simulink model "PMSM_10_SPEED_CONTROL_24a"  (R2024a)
settings: Solver=ode45  StartTime=0.0  StopTime=0.2  MaxStep=1e-6  RelTol=1e-6  AbsTol=1e-6  EnableMultiTasking=on
undefined symbols (not defined in the file): by, established, Flux, linkage, magnets, V
libraries: spsIGBTDiodeLib x6, spsCurrentMeasurementLib x3, slpidlib x2, simulink x2, spsDCVoltageSourceLib x1, spsPermanentMagnetSynchronousMachineLib x1, spspowerguiLib x1

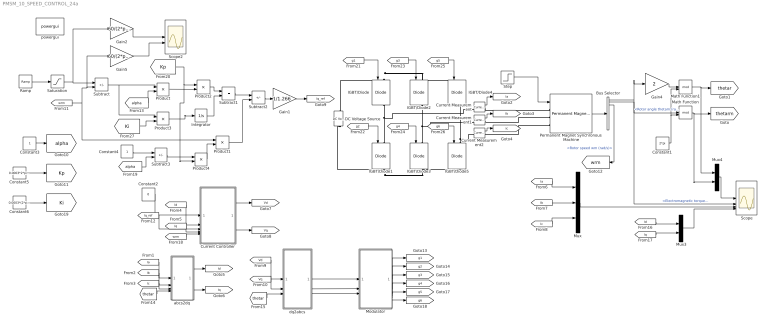
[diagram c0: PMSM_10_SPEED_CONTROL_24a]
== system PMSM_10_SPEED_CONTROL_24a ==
  Bus Selector : BusSelector  OutputSignals=Rotor angle thetam (rad),Electromagnetic torque Te (N*m),Rotor speed wm (rad/s)
  Constant1 : Constant  Value=2*pi
  Constant2 : Constant  Value=0
  Constant3 : Constant
  Constant4 : Constant
  Constant5 : Constant  Value=0.0003*2*pi*50/1.266
  Constant6 : Constant  Value=0.0003*(2*pi*50)^2/1.266/5
  Current Controller : Subsystem
  Current Measurement : spsCurrentMeasurementLib/Current Measurement  PhasorSimulation=off  OutputType=Complex  PSBequivalent=0
  Current Measurement1 : spsCurrentMeasurementLib/Current Measurement  PhasorSimulation=off  OutputType=Complex  PSBequivalent=0
  Current Measurement2 : spsCurrentMeasurementLib/Current Measurement  PhasorSimulation=off  OutputType=Complex  PSBequivalent=0
  DC Voltage Source : spsDCVoltageSourceLib/DC Voltage Source  Amplitude=400  Measurements=None
  Gain1 : Gain  Gain=1/1.266
  Gain2 : Gain  Gain=60/(2*pi)
  Gain4 : Gain  Gain=2
  Gain5 : Gain  Gain=60/(2*pi)
  IGBT/Diode{,1..5} (6 alike) : spsIGBTDiodeLib/IGBT//Diode  Ron=1e-3  Rs=1e5  Cs=inf  Measurements=on
  Integrator : Integrator
  Math Function : Math  Operator=mod  SignedPower=on
  Math Function1 : Math  Operator=mod  SignedPower=on
  Modulator : Subsystem
  Mux : Mux  Inputs=3
  Mux3 : Mux  Inputs=2
  Mux4 : Mux  Inputs=2
  Permanent Magnet Synchronous Machine : spsPermanentMagnetSynchronousMachineLib/Permanent Magnet Synchronous Machine  NbPhases=3  FluxDistribution=Sinusoidal  RotorType=Round  MechanicalLoad=Torque Tm  PresetModel=No  ShowDetailedParameters=on  MeasurementBus=off  Resistance=0.423  Inductance=8.5e-3  dqInductances=[8.5e-3,8.5e-3]  La=0.00476  MachineConstant=Flux linkage established by magnets (V.s)  Flux=0.422  VoltageCst=153.0847  TorqueCst=1.266  Flat=120  Mechanical=[0.0003 0.0 2 0]  PolePairs=2  InitialConditions=[0,0, 0,0]  InitialConditions5ph=[0 0 0 0 0 0]  RefAngle=Aligned with phase A axis (original Park)  IterativeDiscreteModel=Trapezoidal non iterative  TsBlock=-1  TsPowergui=0
  Product{,1..4} (5 alike) : Product
  Ramp : simulink/Sources/Ramp  slope=2000/0.05/60*2*pi  start=0  InitialOutput=0
  Saturation : Saturate  UpperLimit=2000/60*2*pi  LowerLimit=0
  Scope : Scope  NumInputPorts=4
  Scope2 : Scope  NumInputPorts=2
  Step : Step  Time=0.1  Before=1  After=3  SampleTime=0
  Subtract : Sum  Inputs=+-
  Subtract1 : Sum
  Subtract2 : Sum  Inputs=+-
  Subtract3 : Sum  Inputs=+-
  abcs2dq : Subsystem
  dq2abcs : Subsystem
  powergui : spspowerguiLib/powergui  Priority=1  SimulationMode=Continuous  SampleTime=50e-6  frequency=60  Iterations=50  frequencyindice=0  Pbase=100e6  ErrMax=1e-4  UnitsV=kV  UnitsW=MW  buscounter=0  FunctionMessages=off  echomessages=off  EnableUseOfTLC=off  CurrentSourceSwitches=off  DisableSnubberDevices=on  DisableRonSwitches=on  DisableVfSwitches=on  DisplayEquations=off  AutomaticDiscreteSolvers=off  SolverType=Tustin  Interpol=off  ExternalGateDelay=off  methode=off  Ts=0  x0status=blocks  SPID=on  SwTol=0  HookPort=off  NonlinearTolerance=1e-4  nMaxIteration=100  ContinueOnMaxIteration=off  RestoreLinks=warning  ResistiveCurrentMeasurement=off  Frange=[0:2:500]  Ylog=off  Xlog=on  ShowGrid=off  save=off  variable=ZData  structure=0  ZoomFFT=off  StartTime=0.0  cycles=1  DisplayStyle=1  fundamental=60  FreqAxis=off  MaxFrequency=1000  frequencyindicesteady=1  RmsSteady=1  display=off
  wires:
  Step/1 -> Permanent Magnet Synchronous Machine/1
  Permanent Magnet Synchronous Machine/1 -> Bus Selector/1
  Mux/1 -> Scope/3
  Bus Selector/2 -> Scope/2  "<Electromagnetic torque Te (N*m)>"
  Bus Selector/1 -> Gain4/1, Math Function/1  "<Rotor angle thetam (rad)>"
  Constant1/1 -> Math Function1/2, Math Function/2
  Math Function/1 -> Mux4/2, [thetarm]
  Gain4/1 -> Math Function1/1
  Math Function1/1 -> Mux4/1, [thetar]
  [Ia] -> Mux/1
  [Ib] -> Mux/2
  [Ic] -> Mux/3
  Mux3/1 -> Scope/4
  [Id] -> Mux3/1
  [Iq] -> Mux3/2
  Mux4/1 -> Scope/1
  Bus Selector/3 -> [wrm]  "<Rotor speed wm (rad/s)>"
  [g1] -> IGBT/Diode/1
  [g2] -> IGBT/Diode1/1
  [g3] -> IGBT/Diode2/1
  [g4] -> IGBT/Diode3/1
  [g5] -> IGBT/Diode4/1
  [g6] -> IGBT/Diode5/1
  Current Measurement/1 -> [Ia]
  Current Measurement1/1 -> [Ib]
  Current Measurement2/1 -> [Ic]
  Modulator/1(g1) -> [g1]
  Modulator/2(g2) -> [g2]
  Modulator/3(g3) -> [g3]
  Modulator/4(g4) -> [g4]
  Modulator/5(g5) -> [g5]
  Modulator/6(g6) -> [g6]
  Constant2/1 -> Current Controller/1(Id_ref)
  [Id] -> Current Controller/2(Id)
  [Iq_ref] -> Current Controller/3(Iq_ref)
  [Iq] -> Current Controller/4(Iq)
  [wrm] -> Current Controller/5(Wrm)
  Current Controller/1(Vd_ref) -> [Vd]
  Current Controller/2(Vq_ref) -> [Vq]
  [Ia] -> abcs2dq/1(as)
  [Ib] -> abcs2dq/2(bs)
  [Ic] -> abcs2dq/3(cs)
  [thetar] -> abcs2dq/4(thetar)
  abcs2dq/1(d) -> [Id]
  abcs2dq/2(q) -> [Iq]
  [Vd] -> dq2abcs/1(d)
  [Vq] -> dq2abcs/2(q)
  [thetar] -> dq2abcs/3(thetar)
  dq2abcs/3(cs) -> Modulator/3(Vcs_ref)
  dq2abcs/2(bs) -> Modulator/2(Vbs_ref)
  dq2abcs/1(as) -> Modulator/1(Vas_ref)
  Subtract/1 -> Product/1, Product3/1
  [wrm] -> Product1/1, Gain5/1, Subtract/2
  Ramp/1 -> Saturation/1
  Subtract2/1 -> Gain1/1
  Gain1/1 -> [Iq_ref]
  Gain5/1 -> Scope2/2
  Saturation/1 -> Gain2/1, Subtract/1
  Gain2/1 -> Scope2/1
  Product3/1 -> Integrator/1
  Product2/1 -> Subtract1/1
  Constant3/1 -> [alpha]
  Product/1 -> Product2/2
  [alpha] -> Product/2
  Integrator/1 -> Subtract1/2
  Subtract1/1 -> Subtract2/1
  Constant4/1 -> Subtract3/1
  [alpha] -> Subtract3/2
  Subtract3/1 -> Product4/1
  Product4/1 -> Product1/2
  Product1/1 -> Subtract2/2
  Constant5/1 -> [Kp]
  Constant6/1 -> [Ki]
  [Kp] -> Product4/2, Product2/1
  [Ki] -> Product3/2
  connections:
  IGBT/Diode1/LConn1 -- Current Measurement/LConn1 -- IGBT/Diode/RConn1
  IGBT/Diode3/LConn1 -- Current Measurement1/LConn1 -- IGBT/Diode2/RConn1
  IGBT/Diode5/LConn1 -- Current Measurement2/LConn1 -- IGBT/Diode4/RConn1
  DC Voltage Source/RConn1 -- IGBT/Diode4/LConn1 -- IGBT/Diode2/LConn1 -- IGBT/Diode/LConn1
  IGBT/Diode1/RConn1 -- IGBT/Diode5/RConn1 -- IGBT/Diode3/RConn1 -- DC Voltage Source/LConn1
  Current Measurement2/RConn1 -- Permanent Magnet Synchronous Machine/LConn3
  Current Measurement1/RConn1 -- Permanent Magnet Synchronous Machine/LConn2
  Current Measurement/RConn1 -- Permanent Magnet Synchronous Machine/LConn1

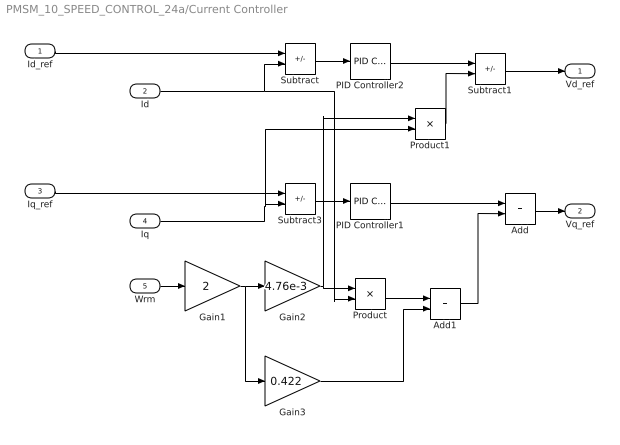
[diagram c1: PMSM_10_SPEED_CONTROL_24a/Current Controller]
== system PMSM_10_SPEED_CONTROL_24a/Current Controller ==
  Id_ref : Inport
  Id : Inport  Port=2
  Iq_ref : Inport  Port=3
  Iq : Inport  Port=4
  Wrm : Inport  Port=5
  Add : Sum
  Add1 : Sum
  Gain1 : Gain  Gain=2
  Gain2 : Gain  Gain=4.76e-3
  Gain3 : Gain  Gain=0.422
  PID Controller1 : slpidlib/PID Controller  Controller=PI  Form=Parallel  TimeDomain=Continuous-time  UseExternalTs=off  SampleTime=1  IntegratorMethod=Forward Euler  FilterMethod=Forward Euler  ControllerParametersSource=internal  P=14.95  I=1328.9  UseKiTs=off  D=0  UseExternalDerivativeSource=off  N=100  UseFilter=on  TunerSelectOption=Transfer Function Based (PID Tuner App)  InitialConditionSource=internal  InitialConditionForIntegrator=0  InitialConditionForFilter=0  DifferentiatorICPrevScaledInput=0  ExternalReset=none  TrackingMode=off  Kt=1  LimitOutput=off  SatLimitsSource=internal  UpperSaturationLimit=inf  LowerSaturationLimit=-inf  LinearizeAsGain=on  AntiWindupMode=none  Kb=1  LimitIntegrator=off  UpperIntegratorSaturationLimit=inf  LowerIntegratorSaturationLimit=-inf  POutMin=[]  POutMax=[]  IOutMin=[]  IOutMax=[]  DOutMin=[]  DOutMax=[]  NOutMin=[]  NOutMax=[]  SumOutMin=[]  SumOutMax=[]  SaturationOutMin=[]  SaturationOutMax=[]  PParamMin=[]  PParamMax=[]  IParamMin=[]  IParamMax=[]  DParamMin=[]  DParamMax=[]  NParamMin=[]  NParamMax=[]  KbParamMin=[]  KbParamMax=[]  KtParamMin=[]  KtParamMax=[]  KbOutMin=[]  KbOutMax=[]  KtOutMin=[]  KtOutMax=[]  IntegratorOutMin=[]  IntegratorOutMax=[]  FilterOutMin=[]  FilterOutMax=[]  SumI1OutMin=[]  SumI1OutMax=[]  SumI2OutMin=[]  SumI2OutMax=[]  SumI3OutMin=[]  SumI3OutMax=[]  SumI4OutMin=[]  SumI4OutMax=[]  SumDOutMin=[]  SumDOutMax=[]  DifferentiatorOutMin=[]  DifferentiatorOutMax=[]  FilterDiffOutCoefMin=[]  FilterDiffOutCoefMax=[]  ReciprocalOutMin=[]  ReciprocalOutMax=[]  SumDenOutMin=[]  SumDenOutMax=[]  SumNumOutMin=[]  SumNumOutMax=[]  DivideOutMin=[]  DivideOutMax=[]  UdiffTsProdOutMin=[]  UdiffTsProdOutMax=[]  NTsProdOutMin=[]  NTsProdOutMax=[]  UintegralTsProdOutMin=[]  UintegralTsProdOutMax=[]  UngainTsProdOutMin=[]  UngainTsProdOutMax=[]  ClampingZeroOutDataTypeStr=Inherit: Inherit via back propagation  ClampingZeroOutMin=[]  ClampingZeroOutMax=[]  FilterDenConstantOutDataTypeStr=Inherit: Inherit via back propagation  FilterDenConstantOutMin=[]  FilterDenConstantOutMax=[]  PCopyOutDataTypeStr=Inherit: Inherit via back propagation  PCopyOutMin=[]  PCopyOutMax=[]  NCopyOutDataTypeStr=Inherit: Inherit via back propagation  NCopyOutMin=[]  NCopyOutMax=[]  IntegratorContinuousStateAttributes=''  IntegratorStateMustResolveToSignalObject=off  IntegratorRTWStateStorageClass=Auto  FilterContinuousStateAttributes=''  FilterStateMustResolveToSignalObject=off  FilterRTWStateStorageClass=Auto  ParallelPVariant=InternalParameters  IdealPVariant=Disabled  IVariant=InternalParameters  DVariant=Disabled  IntegratorVariant=Continuous  SatVariant=Disabled  AWVariant=Passthrough  PCopyVariant=Disabled  TRVariant=Disabled  FdbkBlocksVariant=Forward  IdealPFdbkVariant=Disabled  SatFdbkVariant=Disabled  DerivativeFilterVariant=Disabled  NVariant=Disabled  NCopyVariant=Disabled_SignalSpec  FilterICVariant=Disabled  IntegratorICVariant=InternalICs  ExternalResetVariant=Disabled  TRSumVariant=Passthrough  SumFdbkVariant=Disabled  SumVariant=Sum_PI  TsampFilterVariant=InternalTs  TsampNgainVariant=Passthrough  TsampIntegralVariant=Disabled_SignalSpec  ExternalSaturationOutDataTypeStr=Inherit: Same as second input  DerivativeSourceVariant=Disabled
  PID Controller2 : slpidlib/PID Controller  Controller=PI  Form=Parallel  TimeDomain=Continuous-time  UseExternalTs=off  SampleTime=1  IntegratorMethod=Forward Euler  FilterMethod=Forward Euler  ControllerParametersSource=internal  P=14.95  I=1328.9  UseKiTs=off  D=0  UseExternalDerivativeSource=off  N=100  UseFilter=on  TunerSelectOption=Transfer Function Based (PID Tuner App)  InitialConditionSource=internal  InitialConditionForIntegrator=0  InitialConditionForFilter=0  DifferentiatorICPrevScaledInput=0  ExternalReset=none  TrackingMode=off  Kt=1  LimitOutput=off  SatLimitsSource=internal  UpperSaturationLimit=inf  LowerSaturationLimit=-inf  LinearizeAsGain=on  AntiWindupMode=none  Kb=1  LimitIntegrator=off  UpperIntegratorSaturationLimit=inf  LowerIntegratorSaturationLimit=-inf  POutMin=[]  POutMax=[]  IOutMin=[]  IOutMax=[]  DOutMin=[]  DOutMax=[]  NOutMin=[]  NOutMax=[]  SumOutMin=[]  SumOutMax=[]  SaturationOutMin=[]  SaturationOutMax=[]  PParamMin=[]  PParamMax=[]  IParamMin=[]  IParamMax=[]  DParamMin=[]  DParamMax=[]  NParamMin=[]  NParamMax=[]  KbParamMin=[]  KbParamMax=[]  KtParamMin=[]  KtParamMax=[]  KbOutMin=[]  KbOutMax=[]  KtOutMin=[]  KtOutMax=[]  IntegratorOutMin=[]  IntegratorOutMax=[]  FilterOutMin=[]  FilterOutMax=[]  SumI1OutMin=[]  SumI1OutMax=[]  SumI2OutMin=[]  SumI2OutMax=[]  SumI3OutMin=[]  SumI3OutMax=[]  SumI4OutMin=[]  SumI4OutMax=[]  SumDOutMin=[]  SumDOutMax=[]  DifferentiatorOutMin=[]  DifferentiatorOutMax=[]  FilterDiffOutCoefMin=[]  FilterDiffOutCoefMax=[]  ReciprocalOutMin=[]  ReciprocalOutMax=[]  SumDenOutMin=[]  SumDenOutMax=[]  SumNumOutMin=[]  SumNumOutMax=[]  DivideOutMin=[]  DivideOutMax=[]  UdiffTsProdOutMin=[]  UdiffTsProdOutMax=[]  NTsProdOutMin=[]  NTsProdOutMax=[]  UintegralTsProdOutMin=[]  UintegralTsProdOutMax=[]  UngainTsProdOutMin=[]  UngainTsProdOutMax=[]  ClampingZeroOutDataTypeStr=Inherit: Inherit via back propagation  ClampingZeroOutMin=[]  ClampingZeroOutMax=[]  FilterDenConstantOutDataTypeStr=Inherit: Inherit via back propagation  FilterDenConstantOutMin=[]  FilterDenConstantOutMax=[]  PCopyOutDataTypeStr=Inherit: Inherit via back propagation  PCopyOutMin=[]  PCopyOutMax=[]  NCopyOutDataTypeStr=Inherit: Inherit via back propagation  NCopyOutMin=[]  NCopyOutMax=[]  IntegratorContinuousStateAttributes=''  IntegratorStateMustResolveToSignalObject=off  IntegratorRTWStateStorageClass=Auto  FilterContinuousStateAttributes=''  FilterStateMustResolveToSignalObject=off  FilterRTWStateStorageClass=Auto  ParallelPVariant=InternalParameters  IdealPVariant=Disabled  IVariant=InternalParameters  DVariant=Disabled  IntegratorVariant=Continuous  SatVariant=Disabled  AWVariant=Passthrough  PCopyVariant=Disabled  TRVariant=Disabled  FdbkBlocksVariant=Forward  IdealPFdbkVariant=Disabled  SatFdbkVariant=Disabled  DerivativeFilterVariant=Disabled  NVariant=Disabled  NCopyVariant=Disabled_SignalSpec  FilterICVariant=Disabled  IntegratorICVariant=InternalICs  ExternalResetVariant=Disabled  TRSumVariant=Passthrough  SumFdbkVariant=Disabled  SumVariant=Sum_PI  TsampFilterVariant=InternalTs  TsampNgainVariant=Passthrough  TsampIntegralVariant=Disabled_SignalSpec  ExternalSaturationOutDataTypeStr=Inherit: Same as second input  DerivativeSourceVariant=Disabled
  Product : Product
  Product1 : Product
  Subtract : Sum  Inputs=+-
  Subtract1 : Sum  Inputs=+-
  Subtract3 : Sum  Inputs=+-
  Vd_ref : Outport
  Vq_ref : Outport  Port=2
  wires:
  Add1/1 -> Add/2
  Add/1 -> Vq_ref/1
  Gain1/1 -> Gain3/1, Gain2/1
  Subtract1/1 -> Vd_ref/1
  Iq_ref/1 -> Subtract3/1
  Gain2/1 -> Product1/1, Product/1
  Gain3/1 -> Add1/2
  PID Controller2/1 -> Subtract1/1
  Product1/1 -> Subtract1/2
  Wrm/1 -> Gain1/1
  Product/1 -> Add1/1
  PID Controller1/1 -> Add/1
  Iq/1 -> Product1/2, Subtract3/2
  Id/1 -> Product/2, Subtract/2
  Subtract3/1 -> PID Controller1/1
  Subtract/1 -> PID Controller2/1
  Id_ref/1 -> Subtract/1

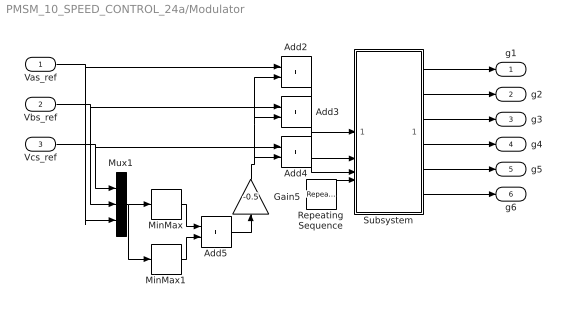
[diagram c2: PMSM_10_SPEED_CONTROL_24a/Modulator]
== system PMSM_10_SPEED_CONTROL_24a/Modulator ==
  Vas_ref : Inport
  Vbs_ref : Inport  Port=2
  Vcs_ref : Inport  Port=3
  Add{2..5} (4 alike) : Sum
  Gain5 : Gain  Gain=-0.5
  MinMax : MinMax
  MinMax1 : MinMax  Function=max
  Mux1 : Mux  Inputs=3
  Repeating Sequence : simulink/Sources/Repeating Sequence  rep_seq_t=[0 0.00005 0.0001]  rep_seq_y=[-200 200 -200]
  Subsystem : Subsystem
  g1 : Outport
  g2 : Outport  Port=2
  g3 : Outport  Port=3
  g4 : Outport  Port=4
  g5 : Outport  Port=5
  g6 : Outport  Port=6
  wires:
  Vcs_ref/1 -> Mux1/1, Add4/1
  MinMax1/1 -> Add5/2
  Gain5/1 -> Add4/2, Add2/2, Add3/2
  Vbs_ref/1 -> Mux1/2, Add3/1
  Add3/1 -> Subsystem/2(Vbn)
  Vas_ref/1 -> Mux1/3, Add2/1
  MinMax/1 -> Add5/1
  Add2/1 -> Subsystem/1(Van)
  Add5/1 -> Gain5/1
  Mux1/1 -> MinMax/1, MinMax1/1
  Add4/1 -> Subsystem/3(Vcn)
  Subsystem/6(g6) -> g6/1
  Subsystem/5(g5) -> g5/1
  Subsystem/4(g4) -> g4/1
  Subsystem/3(g3) -> g3/1
  Subsystem/2(g2) -> g2/1
  Subsystem/1(g1) -> g1/1
  Repeating Sequence/1 -> Subsystem/4(Car)

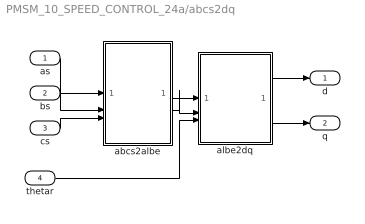
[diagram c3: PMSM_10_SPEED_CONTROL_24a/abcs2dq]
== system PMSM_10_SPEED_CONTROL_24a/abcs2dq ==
  as : Inport
  bs : Inport  Port=2
  cs : Inport  Port=3
  thetar : Inport  Port=4
  abcs2albe : Subsystem
  albe2dq : Subsystem
  d : Outport
  q : Outport  Port=2
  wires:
  albe2dq/1(d) -> d/1
  as/1 -> abcs2albe/1(as)
  abcs2albe/1(alpha) -> albe2dq/1(alpha)
  albe2dq/2(q) -> q/1
  bs/1 -> abcs2albe/2(bs)
  cs/1 -> abcs2albe/3(cs)
  abcs2albe/2(beta) -> albe2dq/2(beta)
  thetar/1 -> albe2dq/3(thetar)

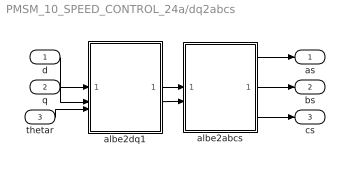
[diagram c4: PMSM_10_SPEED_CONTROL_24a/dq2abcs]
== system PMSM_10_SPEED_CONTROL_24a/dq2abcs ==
  d : Inport
  q : Inport  Port=2
  thetar : Inport  Port=3
  albe2abcs : Subsystem
  albe2dq1 : Subsystem
  as : Outport
  bs : Outport  Port=2
  cs : Outport  Port=3
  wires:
  d/1 -> albe2dq1/1(d)
  q/1 -> albe2dq1/2(q)
  albe2abcs/3(cs) -> cs/1
  thetar/1 -> albe2dq1/3(thetar)
  albe2dq1/2(beta) -> albe2abcs/2(beta)
  albe2abcs/2(bs) -> bs/1
  albe2abcs/1(as) -> as/1
  albe2dq1/1(alpha) -> albe2abcs/1(alpha)

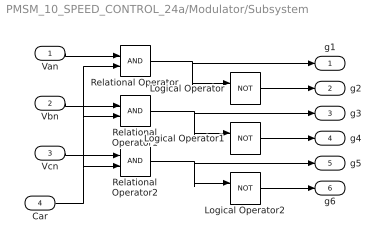
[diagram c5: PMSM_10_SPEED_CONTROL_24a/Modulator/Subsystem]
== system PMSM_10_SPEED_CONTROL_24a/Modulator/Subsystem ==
  Van : Inport
  Vbn : Inport  Port=2
  Vcn : Inport  Port=3
  Car : Inport  Port=4
  Logical Operator : Logic  Operator=NOT  AllPortsSameDT=off  OutDataTypeStr=boolean
  Logical Operator1 : Logic  Operator=NOT  AllPortsSameDT=off  OutDataTypeStr=boolean
  Logical Operator2 : Logic  Operator=NOT  AllPortsSameDT=off  OutDataTypeStr=boolean
  Relational Operator : RelationalOperator  OutDataTypeStr=boolean
  Relational Operator1 : RelationalOperator  OutDataTypeStr=boolean
  Relational Operator2 : RelationalOperator  OutDataTypeStr=boolean
  g1 : Outport
  g2 : Outport  Port=2
  g3 : Outport  Port=3
  g4 : Outport  Port=4
  g5 : Outport  Port=5
  g6 : Outport  Port=6
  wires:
  Relational Operator2/1 -> g5/1, Logical Operator2/1
  Relational Operator1/1 -> g3/1, Logical Operator1/1
  Relational Operator/1 -> g1/1, Logical Operator/1
  Logical Operator2/1 -> g6/1
  Logical Operator1/1 -> g4/1
  Logical Operator/1 -> g2/1
  Car/1 -> Relational Operator/2, Relational Operator1/2, Relational Operator2/2
  Vcn/1 -> Relational Operator2/1
  Vbn/1 -> Relational Operator1/1
  Van/1 -> Relational Operator/1

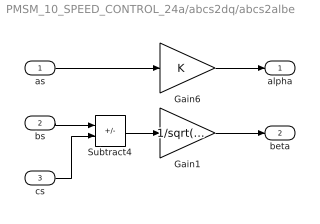
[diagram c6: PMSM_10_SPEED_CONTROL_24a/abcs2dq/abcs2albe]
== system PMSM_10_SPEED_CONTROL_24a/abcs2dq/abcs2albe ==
  as : Inport
  bs : Inport  Port=2
  cs : Inport  Port=3
  Gain1 : Gain  Gain=1/sqrt(3)
  Gain6 : Gain
  Subtract4 : Sum  Inputs=+-
  alpha : Outport
  beta : Outport  Port=2
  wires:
  bs/1 -> Subtract4/1
  as/1 -> Gain6/1
  cs/1 -> Subtract4/2
  Gain1/1 -> beta/1
  Subtract4/1 -> Gain1/1
  Gain6/1 -> alpha/1

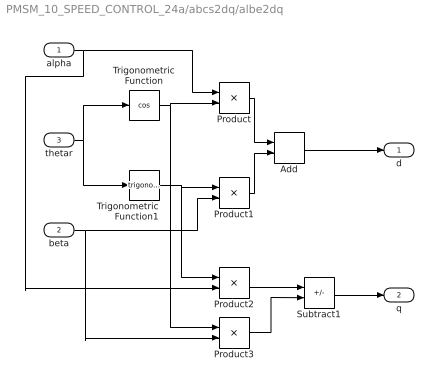
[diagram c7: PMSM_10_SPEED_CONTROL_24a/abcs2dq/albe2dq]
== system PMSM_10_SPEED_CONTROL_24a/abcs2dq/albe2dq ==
  alpha : Inport
  beta : Inport  Port=2
  thetar : Inport  Port=3
  Add : Sum
  Product{,1..3} (4 alike) : Product
  Subtract1 : Sum  Inputs=-+
  Trigonometric Function : Trigonometry  Operator=cos
  Trigonometric Function1 : Trigonometry
  d : Outport
  q : Outport  Port=2
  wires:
  thetar/1 -> Trigonometric Function/1, Trigonometric Function1/1
  Trigonometric Function/1 -> Product3/1, Product/2
  Trigonometric Function1/1 -> Product2/1, Product1/1
  beta/1 -> Product3/2, Product1/2
  Product/1 -> Add/1
  Product1/1 -> Add/2
  Add/1 -> d/1
  Subtract1/1 -> q/1
  alpha/1 -> Product/1, Product2/2
  Product2/1 -> Subtract1/1
  Product3/1 -> Subtract1/2

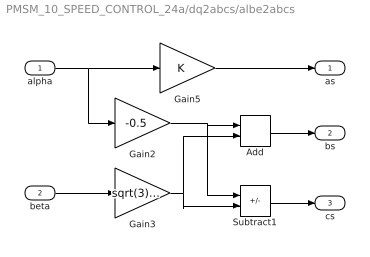
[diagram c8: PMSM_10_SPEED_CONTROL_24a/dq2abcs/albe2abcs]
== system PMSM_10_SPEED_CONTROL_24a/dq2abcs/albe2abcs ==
  alpha : Inport
  beta : Inport  Port=2
  Add : Sum
  Gain2 : Gain  Gain=-0.5
  Gain3 : Gain  Gain=sqrt(3)/2
  Gain5 : Gain
  Subtract1 : Sum  Inputs=+-
  as : Outport
  bs : Outport  Port=2
  cs : Outport  Port=3
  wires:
  alpha/1 -> Gain2/1, Gain5/1
  Gain3/1 -> Subtract1/2, Add/2
  Gain2/1 -> Subtract1/1, Add/1
  Add/1 -> bs/1
  Subtract1/1 -> cs/1
  beta/1 -> Gain3/1
  Gain5/1 -> as/1

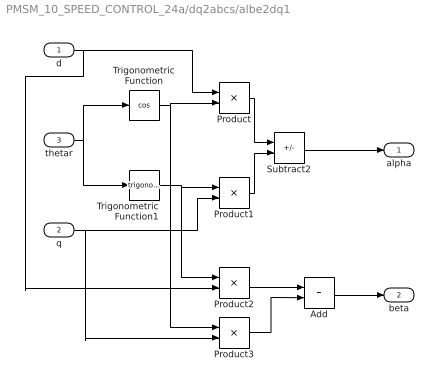
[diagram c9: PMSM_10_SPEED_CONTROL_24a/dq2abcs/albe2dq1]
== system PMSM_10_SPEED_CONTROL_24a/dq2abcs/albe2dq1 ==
  d : Inport
  q : Inport  Port=2
  thetar : Inport  Port=3
  Add : Sum
  Product{,1..3} (4 alike) : Product
  Subtract2 : Sum  Inputs=+-
  Trigonometric Function : Trigonometry  Operator=cos
  Trigonometric Function1 : Trigonometry
  alpha : Outport
  beta : Outport  Port=2
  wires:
  Product3/1 -> Add/2
  Product2/1 -> Add/1
  d/1 -> Product2/2, Product/1
  Add/1 -> beta/1
  Subtract2/1 -> alpha/1
  Product1/1 -> Subtract2/2
  Product/1 -> Subtract2/1
  q/1 -> Product1/2, Product3/2
  Trigonometric Function1/1 -> Product1/1, Product2/1
  Trigonometric Function/1 -> Product/2, Product3/1
  thetar/1 -> Trigonometric Function1/1, Trigonometric Function/1
